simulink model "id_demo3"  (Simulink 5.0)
settings: Solver=ode45  SolverMode=SingleTasking  StartTime=0.0  StopTime=10  RelTol=1e-3  AbsTol=1e-3

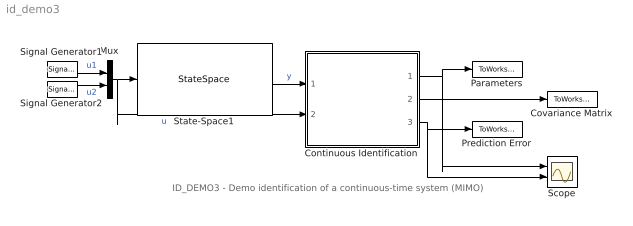
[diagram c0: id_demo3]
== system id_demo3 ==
  note: ID_DEMO3 - Demo identification of a continuous-time system (MIMO)
  Continuous Identification : Subsystem  mask(Continuous Identification){par3=[2,2], par1=[0,1], tc=[1], par2=[0.985,0.01], poc=[0 0 0 0 0 0 0 0], kov=[10e6], ts=[1]}
      mask prompts: par3 "Number of inputs and outputs -  [in,out]:"; par1 "Degrees of numerator and denominator -  [dn, dd]:"; tc "Time constant of the filter - [Tc]:"; par2 "Exponential forgetting and Bittanti's correction - [L, d]:"; poc "Initial parameter estimates - [theta(1) ... theta(n)]:"; kov "Covariance matrix (see help, standard - [10e6]):"; ts "Sampling time - [ts]:"
      mask help: Continuous identification Authors: Lubos Cirka and Miroslav Fikar 1998 - 2006
      mask init:
      | % State-space realisation of continuous-time filters
      | %
      | % Input:
      | %    y_1(t), ..., y_in(t), u_1(t), ..., u_out(t)
      | % Output:
      | %    y_1(t), ..., y_in(t), -y_1'(t), ..., -y_in'(t), -y_1''(t), ..., -y_in''(t), ..., 
      | %    u_1(t), ..., u_out(t), u_1'(t), ..., u_out'(t), u_1''(t), ..., u_out''(t), ...
      | 
      | % Parameters definition
      | cit = par1(1); % numerator degree 
      | men = par1(2); % denumerator degree
      | L = par2(1); % exponential forgetting
      | d = par2(2); % Bittanti's correction
      | n = (cit+1)*par3(1)+men*par3(2); % number of data
      | m = par3(2); % 
      | in = par3(1); % number of inputs
      | out = par3(2); % number of outputs
      | 
      | % Calculation of the denominator with multiple time constant tc
      | den = 1;
      | for i = 1:men,
      |    den = conv([tc 1],den);
      | end;
      | a = fliplr(den(2:men+1)/den(1));
      | 
      | % State-space realisation of the output filter ([Ay, By, Cy, Dy])
      | A0 = zeros(out*(men-1),out);
      | A1 = eye(out*(men-1));
      | for i = 1:men
      |    A2(1:out,out*(i-1)+1:i*out) = -a(i)*eye(out);
      | end
      | Ay = [A0 A1;A2];
      | B0 = zeros(out*(men-1),out);
      | B1 = eye(out,out);
      | By = [B0;B1];
      | 
      | C0 = -eye(out*(men-1)+out);
      | C0(1:out,1:out) = eye(out);
      | for i = 1:men
      |    C1(1:out,out*(i-1)+1:i*out) = a(i)*eye(out);
      | end
      | Cy = [C0;C1]/den(1);
      | Dy = -[zeros(out,out);By]/den(1);
      | 
      | % State-space realisation of the input filter ([Au, Bu, Cu, Du])
      | a0 = zeros(in*(men-1),in);
      | a1 = eye(in*(men-1));
      | for i = 1:men
      |    a2(1:in,in*(i-1)+1:i*in) = -a(i)*eye(in);
      | end
      | Au = [a0 a1;a2];
      | b0 = zeros(in*(men-1),in);
      | b1 = eye(in,in);
      | Bu = [b0;b1];
      | if cit==men
      |    c0 = eye(in*(cit-1)+in);
      |    for i = 1:cit
      |       c1(1:in,in*(i-1)+1:i*in) = -a(i)*eye(in);
      |    end
      |    Cu = [c0;c1]/den(1);
      |    Du = [zeros(in*(cit-1)+in,in);eye(in)]/den(1);
      | else
      |    c0 = eye(in*(cit+1));
      |    c1 = zeros(in*(cit+1),(men-cit-1)*in);
      |    Cu = [c0 c1]/den(1);
      |    Du = zeros(in*(cit+1),in);
      | end
  Covariance Matrix : ToWorkspace  VariableName=CovMatrix  SaveFormat=Array
  Mux : Mux  Inputs=2
  Parameters : ToWorkspace  VariableName=AB  SaveFormat=Array
  Prediction Error : ToWorkspace  VariableName=PredError  SaveFormat=Array
  Scope : Scope  NumInputPorts=2
  Signal Generator1 : SignalGenerator  Units=rad/sec
  Signal Generator2 : SignalGenerator  WaveForm=square  Frequency=2  Units=rad/sec
  State-Space1 : StateSpace  A=[-23 30;15 -20]  B=[1 1.3;1.1 2.1]  C=[23 -30;-15 20]  D=[0 0;0 0]
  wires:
  State-Space1/1 -> Continuous Identification/1(y)  "y"
  Mux/1 -> State-Space1/1, Continuous Identification/2(u)  "u"
  Continuous Identification/1(B) -> Scope/1, Parameters/1
  Continuous Identification/2("Covariance matrix ") -> Covariance Matrix/1
  Continuous Identification/3(prediction error) -> Prediction Error/1, Scope/2
  Signal Generator1/1 -> Mux/1  "u1"
  Signal Generator2/1 -> Mux/2  "u2"

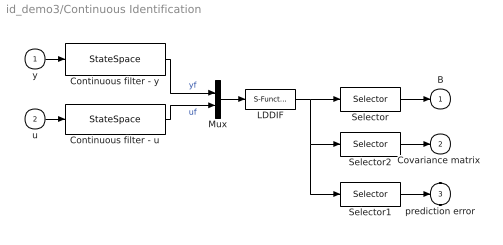
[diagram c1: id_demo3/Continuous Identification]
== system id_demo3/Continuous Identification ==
  y : Inport
  u : Inport  Port=2
  Continuous filter - u : StateSpace  A=Au  B=Bu  C=Cu  D=Du
  Continuous filter - y : StateSpace  A=Ay  B=By  C=Cy  D=Dy
  LDDIF : S-Function  FunctionName=lddif_s  Parameters=m, n, L, d, poc, kov, ts
  Mux : Mux  Inputs=2
  Selector : Selector  Elements=[1:1:n*m]  InputPortWidth=n*m+n*n+m
  Selector1 : Selector  Elements=[n*m+n*n+1:1:n*m+n*n+m]  InputPortWidth=n*m+n*n+m
  Selector2 : Selector  Elements=[n*m+1:1:n*m+n*n]  InputPortWidth=n*m+n*n+m
  B : Outport  InitialOutput=0
  "Covariance matrix " : Outport  Port=2  InitialOutput=0
  prediction error : Outport  Port=3  InitialOutput=0
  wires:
  Continuous filter - u/1 -> Mux/2  "uf"
  Continuous filter - y/1 -> Mux/1  "yf"
  u/1 -> Continuous filter - u/1
  y/1 -> Continuous filter - y/1
  Mux/1 -> LDDIF/1
  LDDIF/1 -> Selector2/1, Selector1/1, Selector/1
  Selector/1 -> B/1
  Selector2/1 -> "Covariance matrix "/1
  Selector1/1 -> prediction error/1
